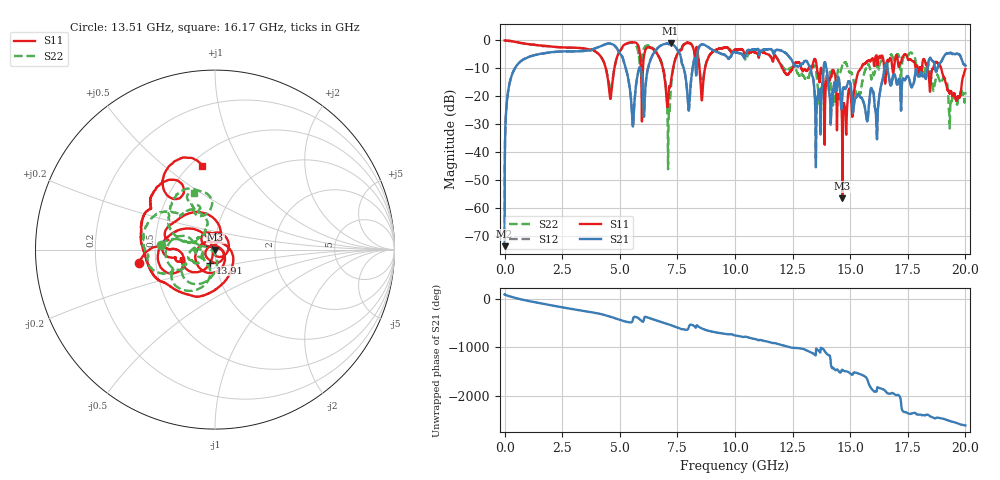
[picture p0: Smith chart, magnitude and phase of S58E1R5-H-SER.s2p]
!{S58E1R5}
!Johanson Technology Inc.
!www.johansontechnology.com
!Test Board Conditions:
!Substrate Type  RO4350B
!Substrate Thickness  60 mil
!Substrate Dk  3.66
!TL Type: GCPW
!TL Trace Width  115 mil
!TL Gap  52 mil
!Electrode orientation  Horizontal
!DUT TOPOLOGY	SERIES
!Mounting Pad LxW  55x428 mil
! Created Tue Apr 13 22:22:31 2021
# hz S ma R 50
! 2 Port Network Data from SP1.SP block
! freq  magS11  angS11  magS21  angS21  magS12  angS12  magS22  angS22
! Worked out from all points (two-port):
!   20001 points, 300 kHz to 20 GHz, reference 50 ohm
!   highest |S21| = -1.02 dB at 7.203 GHz (marker M1); lowest = -73.7 dB at 300 kHz (marker M2)
!   |S21| within 3 dB of the highest: 2.31 GHz to 4.962 GHz (2.652 GHz wide, 72.9 % of centre); 6.515 GHz to 7.545 GHz (1.03 GHz wide, 14.7 % of centre)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
!   lowest |S11| = -56.5 dB at 14.66 GHz (marker M3), VSWR 1.00, Z = 50.1 - j0.122 ohm
!   |S11| at or under -10 dB: 12.06 GHz to 12.51 GHz (450.8 MHz wide, 3.67 % of centre); 13.75 GHz to 15.46 GHz (1.711 GHz wide, 11.7 % of centre); 18.95 GHz to end of sweep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
!   |S22| runs from -46.1 to 0.0 dB; largest |S21 - S12| = 0.01
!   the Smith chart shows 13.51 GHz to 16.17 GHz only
!   S11 on the Smith chart (normalised r, x): 13.51 GHz: 0.40, -0.08; 13.91 GHz: 0.94, -0.14; 16.17 GHz: 0.57, +0.68
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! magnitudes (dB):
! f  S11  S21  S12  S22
! 300 kHz  0.0  -73.7  -70.0  0.0
! 126.3 MHz  -0.1  -19.8  -19.8  -0.1
! 452.3 MHz  -0.5  -9.9  -9.9  -0.5
! 3.334 GHz  -2.8  -3.8  -3.8  -2.8
! 4.593 GHz  -20.9  -1.1  -1.1  -18.4
! 5.564 GHz  -0.6  -30.8  -30.8  -0.9
! 5.963 GHz  -27.3  -13.4  -13.4  -6.1
! 6.667 GHz  -5.4  -2.6  -2.5  -5.2
! 7.203 GHz  -15.7  -1.0  -1.0  -18.5
! 7.984 GHz  -0.9  -24.9  -24.8  -0.9
! 8.57 GHz  -21.0  -1.4  -1.4  -17.0
! 10 GHz  -3.2  -4.2  -4.2  -3.5
! 13.33 GHz  -9.8  -12.2  -12.0  -9.1
! 13.51 GHz  -7.4  -42.3  -39.6  -10.3
! 13.91 GHz  -22.3  -7.9  -8.0  -17.9
! 14.28 GHz  -10.9  -17.3  -17.2  -20.4
! 14.66 GHz  -56.5  -19.0  -18.9  -8.7
! 15.35 GHz  -11.3  -19.2  -19.3  -19.0
! 16.17 GHz  -6.5  -33.8  -33.5  -9.4
! 16.67 GHz  -7.5  -12.5  -12.6  -6.4
! 19.66 GHz  -20.6  -4.8  -4.8  -22.3
! 20 GHz  -10.3  -9.1  -9.1  -18.5
